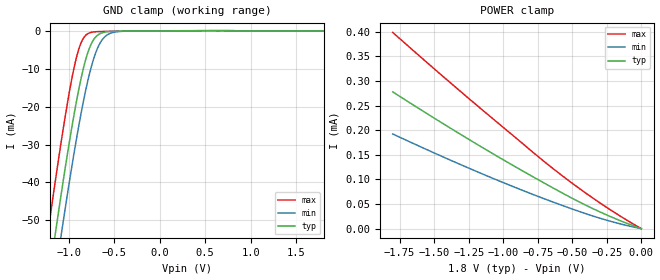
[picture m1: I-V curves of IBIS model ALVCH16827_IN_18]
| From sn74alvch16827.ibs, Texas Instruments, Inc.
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[Model]   ALVCH16827_IN_18
Model_type  Input
Vinl=0.5775
Vinh=1.2675
| variable   typ   min   max
C_comp   0.93pF   0.71pF   1.10pF
[Temperature Range]   40   100   -40
| Ambient temperature   25   85   -40
[Voltage range]   1.8   1.65   1.95
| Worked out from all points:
|   GND clamp passes 1 mA (typ) near -0.67 V on its own axis
[GND Clamp]
| ALVCH16827_IN_18
|   Voltage   I(typ)   I(min)   I(max)
-1.8V     -169.9mA   -179.9mA   -157.2mA
-1.22V    -66.14mA   -76.92mA   -52.29mA
-1.14V    -52.75mA   -63.55mA   -38.86mA
-1.075V   -42.25mA   -53mA      -28.45mA
-935mV    -21.51mA   -31.66mA   -9.294mA
-860mV    -12.31mA   -21.51mA   -3.028mA
-785mV    -5.515mA   -12.83mA   -697.5uA
-725mV    -2.335mA   -7.435mA   -280.9uA
-660mV    -800.2uA   -3.497mA   -176.2uA
-590mV    -269.6uA   -1.316mA   -141.1uA
-495mV    -100.9uA   -318.8uA   -112.5uA
1.8V      1.113nA    9.574uA    -22.72uA
[POWER Clamp]
| ALVCH16827_IN_18
|   Voltage   I(typ)   I(min)   I(max)
-1.8V     278uA      192.5uA    398.9uA
-1.2V     173.2uA    117.1uA    252.9uA
-645mV    83.65uA    54.66uA    123.4uA
-480mV    58.73uA    37.93uA    88.08uA
-315mV    36.04uA    22.58uA    55.28uA
-155mV    16.49uA    9.93uA     25.95uA
-16.28fV  1.113nA    59.61nA    5.251pA
